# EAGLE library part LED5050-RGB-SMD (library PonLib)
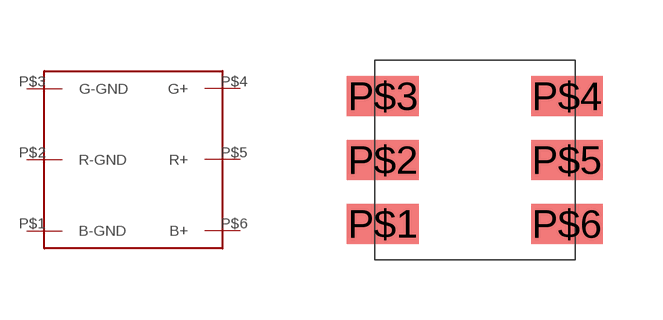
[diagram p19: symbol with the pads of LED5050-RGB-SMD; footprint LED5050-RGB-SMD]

Designator prefix -

## LED5050-RGB-SMD  [LED5050-RGB-SMD]
P$1  B-GND
P$2  R-GND
P$3  G-GND
P$4  G+
P$5  R+
P$6  B+

## Footprint LED5050-RGB-SMD (pad centres in mm)
smd 1.8 x 1: P$1 -2.3,-1.6; P$2 -2.3,0; P$3 -2.3,1.6; P$4 2.3,1.6; P$5 2.3,0; P$6 2.3,-1.6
